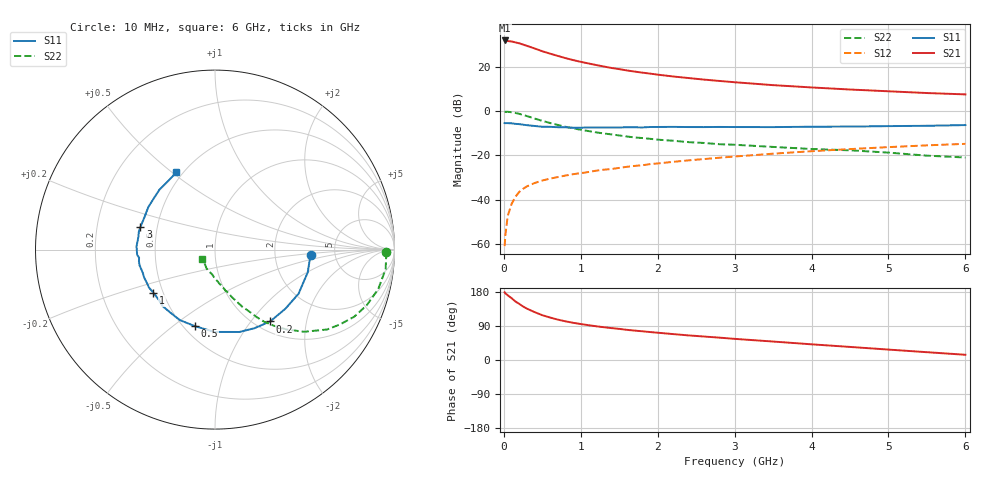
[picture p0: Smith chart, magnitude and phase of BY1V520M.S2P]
! SIEMENS Small Signal Semiconductors
! BFY420
! Si NPN RF SIEGET Grounded Emitter Transistor in MICRO-X
! VCE = 1.5 V  IC = 20 mA
! Common Emitter S-Parameters:  October  1996
# GHz  S  MA  R  50
!  f  S11  S21  S12  S22
! GHz  MAG  ANG  MAG  ANG  MAG  ANG  MAG  ANG
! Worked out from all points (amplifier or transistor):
!   36 points, 10 MHz to 6 GHz, reference 50 ohm
!   highest |S21| = 31.8 dB at 10 MHz (marker M1)
!   |S21| within 3 dB of that: start of sweep to 348.6 MHz
!   unconditionally stable (mu >= 1): 1.796 GHz to 1.816 GHz; 1.925 GHz to end of sweep
!   at 250 MHz: K = 0.30, MSG = 32.5 dB, |S12| = -35.1 dB
!   at 1.4 GHz: K = 0.93, MSG = 22.8 dB, |S12| = -26.2 dB
!   at 6 GHz: K = 1.08, MAG = 9.4 dB, |S12| = -14.8 dB
!   S11 on the Smith chart (normalised r, x): 10 MHz: 3.26, -0.28; 200 MHz: 1.16, -1.25; 500 MHz: 0.57, -0.60; 1 GHz: 0.44, -0.26; 3 GHz: 0.40, +0.12; 6 GHz: 0.46, +0.52
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0.01  0.5335 -3.3  38.7 178.7  0.0009 104.6  0.9539 -0.8
0.02  0.5311 -5.7  38.37 175.8  0.0016 89.8  0.9544 -2.2
0.1  0.5265 -27.9  36.73 163.2  0.008 80.4  0.9357 -13.6
0.15  0.5121 -40.1  34.99 154.6  0.0116 73.0  0.9008 -20.1
0.2  0.5047 -52.5  33.38 148.1  0.015 71.0  0.8606 -25.8
0.25  0.4899 -63.4  31.26 141.2  0.0176 66.1  0.8107 -31.0
0.3  0.4784 -73.6  29.29 135.5  0.02 65.0  0.7666 -35.5
0.4  0.4587 -90.4  25.54 126.4  0.0238 60.2  0.6751 -42.7
0.5  0.441 -104.6  22.11 118.2  0.0271 58.1  0.5979 -48.1
0.6  0.4389 -116.5  19.56 112.1  0.0299 56.5  0.536 -52.3
0.7  0.4305 -125.0  17.39 106.6  0.0324 55.8  0.4848 -55.8
0.8  0.4294 -132.9  15.51 102.1  0.035 55.0  0.4406 -58.4
1  0.4191 -144.9  12.77 94.9  0.0397 55.1  0.3773 -62.3
1.1  0.4243 -150.2  11.75 91.8  0.0421 55.1  0.3523 -64.5
1.4  0.4226 -162.1  9.29 84.2  0.0492 55.9  0.2961 -68.9
1.6  0.4294 -168.1  8.17 79.6  0.0552 55.7  0.2656 -71.7
2.2  0.4376 177.5  5.977 68.4  0.0714 53.9  0.2134 -78.8
3  0.4341 163.2  4.434 55.8  0.0941 49.8  0.1732 -86.6
3.5  0.4326 155.0  3.814 48.7  0.109 46.6  0.1548 -91.9
4.5  0.4447 140.0  3.038 34.5  0.1384 38.0  0.1298 -102.5
5.5  0.4629 124.3  2.532 20.6  0.1679 28.6  0.0984 -124.9
6  0.4809 116.7  2.36 13.8  0.1816 23.6  0.0894 -142.2
